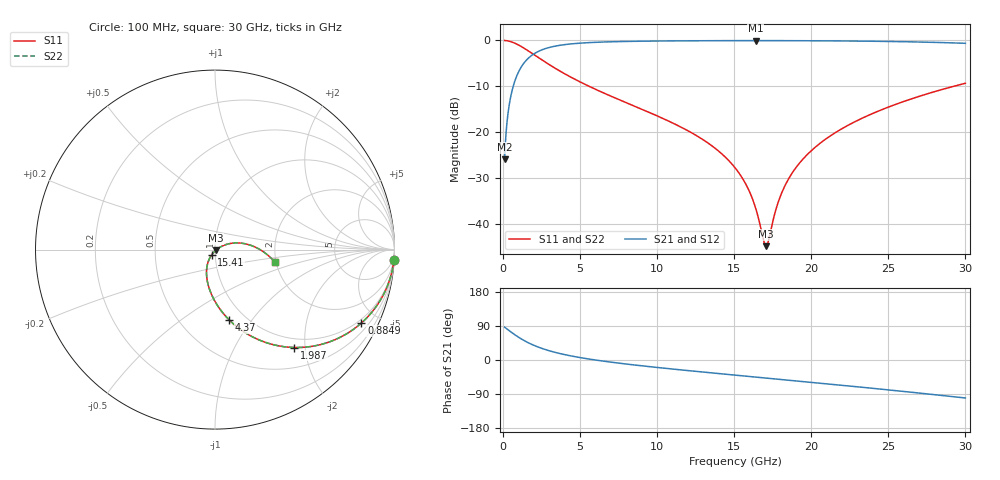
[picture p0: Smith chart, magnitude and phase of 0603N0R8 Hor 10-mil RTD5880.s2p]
# GHz S MA R 50
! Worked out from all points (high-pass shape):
!   3201 points, 100 MHz to 30 GHz, reference 50 ohm
!   highest |S21| = -0.05 dB at 16.39 GHz (marker M1); lowest = -25.9 dB at 100 MHz (marker M2)
!   |S21| within 3 dB of the highest: 1.951 GHz to end of sweep
!   lowest |S11| = -44.9 dB at 17.07 GHz (marker M3), VSWR 1.01, Z = 50.4 - j0.424 ohm
!   |S11| at or under -10 dB: 5.573 GHz to 29.26 GHz (23.68 GHz wide, 136 % of centre)
!   |S22| runs from -44.9 to 0.0 dB; largest |S21 - S12| = 0
!   S11 on the Smith chart (normalised r, x): 100 MHz: 1, -36; 884.9 MHz: 0.83, -4.06; 1.987 GHz: 0.83, -1.79; 4.37 GHz: 0.84, -0.78; 15.41 GHz: 0.96, -0.06; 30 GHz: 1.97, -0.31
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0.1  0.9986 -3.2  0.05059 86.7  0.05059 86.7  0.9986 -3.2
0.436375  0.9762 -13.7  0.2154 76.2  0.2154 76.2  0.9762 -13.7
0.884875  0.9123 -26.6  0.4086 63.3  0.4086 63.3  0.9123 -26.6
1.389438  0.817 -39.1  0.5756 50.8  0.5756 50.8  0.817 -39.1
1.987437  0.7024 -51.0  0.7104 38.9  0.7104 38.9  0.7024 -51.0
3.043281  0.538 -66.0  0.8411 23.8  0.8411 23.8  0.538 -66.0
4.370094  0.3997 -78.6  0.9143 11.1  0.9143 11.1  0.3997 -78.6
5.089563  0.3463 -83.9  0.9355 5.7  0.9355 5.7  0.3463 -83.9
10.06978  0.1484 -108.5  0.9849 -20.0  0.9849 -20.0  0.1484 -108.5
13.12519  0.0795 -119.0  0.992 -32.4  0.992 -32.4  0.0795 -119.0
15.05  0.04084 -122.6  0.9938 -39.9  0.9938 -39.9  0.04084 -122.6
15.40506  0.03385 -122.3  0.994 -41.2  0.994 -41.2  0.03385 -122.3
16.38616  0.01486 -113.2  0.9942 -45.0  0.9942 -45.0  0.01486 -113.2
16.90006  0.006605 -78.2  0.9941 -47.0  0.9941 -47.0  0.006605 -78.2
17.06825  0.005692 -47.7  0.9941 -47.6  0.9941 -47.6  0.005692 -47.7
17.22709  0.006584 -18.8  0.994 -48.2  0.994 -48.2  0.006584 -18.8
17.80641  0.01626 18.3  0.9937 -50.4  0.9937 -50.4  0.01626 18.3
18.28294  0.02581 24.2  0.9934 -52.3  0.9934 -52.3  0.02581 24.2
20.03956  0.0635 25.1  0.9912 -59.0  0.9912 -59.0  0.0635 25.1
22.13256  0.1124 19.1  0.9862 -67.3  0.9862 -67.3  0.1124 19.1
25.01978  0.1878 8.6  0.9738 -78.9  0.9738 -78.9  0.1878 8.6
30  0.3408 -11.9  0.9301 -100.2  0.9301 -100.2  0.3408 -11.9
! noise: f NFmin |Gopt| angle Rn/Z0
0.1  0.003089  0.992  0.3229  0.08896
3.417  0.004122  0.8141  10.47  0.004593
6.743  0.006814  0.7826  19.68  0.006248
10.06  0.009294  0.7662  28.83  0.00759
13.39  0.0117  0.7568  37.85  0.008729
16.7  0.01411  0.7521  46.65  0.00972
20.03  0.0166  0.7509  55.24  0.0106
23.35  0.0192  0.7525  63.57  0.0114
26.67  0.02199  0.7563  71.67  0.01211
30  0.02502  0.762  79.53  0.01276
